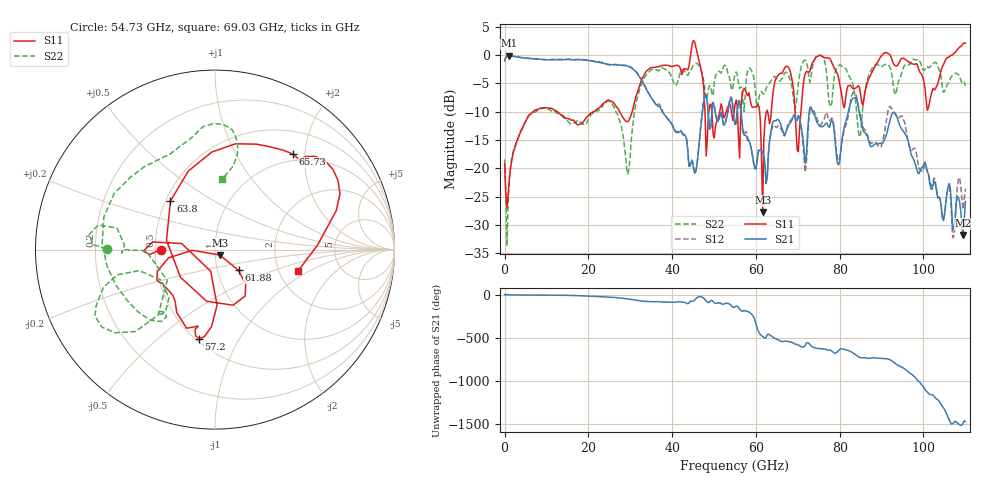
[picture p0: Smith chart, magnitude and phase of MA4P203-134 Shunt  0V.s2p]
!Keysight Technologies,N5247B,US61255204,A.15.70.20
!Date: Friday, October 21, 2022 15:18:02
!Correction: S11(C  4-Port  )
!S31(C  4-Port  )
!S13(C  4-Port  )
!S33(C  4-Port  )
!S2P File: Measurements: S11, S31, S13, S33:
# Hz S  dB  R 50
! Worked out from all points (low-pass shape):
!   401 points, 10 MHz to 110 GHz, reference 50 ohm
!   highest |S21| = -0.16 dB at 1.11 GHz (marker M1); lowest = -31.8 dB at 109.5 GHz (marker M2)
!   |S21| within 3 dB of the highest: start of sweep to 31.56 GHz
!   lowest |S11| = -27.8 dB at 61.6 GHz (marker M3), VSWR 1.09, Z = 52.7 - j3.23 ohm
!   |S11| at or under -10 dB: start of sweep to 6.834 GHz; 12.55 GHz to 21.38 GHz (8.831 GHz wide, 52.1 % of centre); 27.44 GHz to 30.45 GHz (3.015 GHz wide, 10.4 % of centre)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
!   |S22| runs from -33.8 to -0.1 dB; largest |S21 - S12| = 0.16
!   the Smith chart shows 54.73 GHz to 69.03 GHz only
!   S11 on the Smith chart (normalised r, x): 54.73 GHz: 0.54, +0.00; 57.2 GHz: 0.52, -0.69; 61.88 GHz: 1.26, -0.30; 63.8 GHz: 0.53, +0.33; 65.73 GHz: 0.87, +1.76; 69.03 GHz: 2.54, -0.79
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1e7  -19.29 1.8  -1.08 -0.1  -1.09 -0.0  -18.46 -0.5
1.1099e9  -22.26 71.2  -0.16 -0.2  -0.13 -0.2  -22.00 104.3
1.843332e10  -12.13 89.8  -0.87 -11.9  -0.81 -11.8  -11.94 73.9
2.943232e10  -11.75 126.8  -1.99 -47.9  -1.92 -47.0  -21.02 120.9
3.685665e10  -2.07 176.1  -9.07 -80.0  -8.67 -78.7  -2.80 -177.9
4.538088e10  2.25 92.7  -20.88 -60.5  -20.84 -61.2  -1.59 142.4
4.813062e10  -17.85 59.8  -7.12 -71.6  -6.90 -72.2  -7.83 119.7
5.473002e10  -10.38 180.0  -10.98 -147.2  -11.09 -149.3  -4.38 179.6
5.5005e10  -8.75 -175.7  -12.27 -140.7  -12.52 -142.5  -3.33 177.6
5.72048e10  -5.93 -100.1  -14.18 175.8  -14.06 -175.9  -9.99 -147.2
6.16044e10  -27.76 -48.4  -17.32 -124.8  -17.39 -123.1  -6.74 -131.6
6.187938e10  -15.16 -41.4  -17.61 -133.9  -17.73 -132.1  -6.97 -128.9
6.38042e10  -8.69 132.4  -12.55 -122.7  -13.02 -121.4  -4.31 -171.5
6.572902e10  -3.26 50.9  -11.88 -175.2  -12.79 -166.1  -4.60 114.9
6.902872e10  -6.43 -14.6  -10.59 156.7  -10.65 150.6  -8.10 84.2
7.342832e10  -1.52 -176.0  -9.87 116.2  -9.78 111.5  -2.34 158.7
8.085265e10  -8.90 -104.4  -13.60 88.3  -14.00 87.4  -2.12 -129.6
9.185165e10  0.13 89.1  -12.02 -31.8  -9.07 -24.2  -1.99 76.4
9.79011e10  -1.70 174.4  -18.96 123.9  -16.42 122.2  -0.84 -176.2
1.023007e11  -5.91 -68.9  -22.83 -88.9  -22.22 -82.1  -1.47 -114.5
1.0945e11  2.01 39.4  -31.82 -51.2  -27.26 -46.6  -5.00 2.3
1.1e11  2.06 46.4  -25.85 -32.1  -23.61 -30.7  -5.45 11.4
